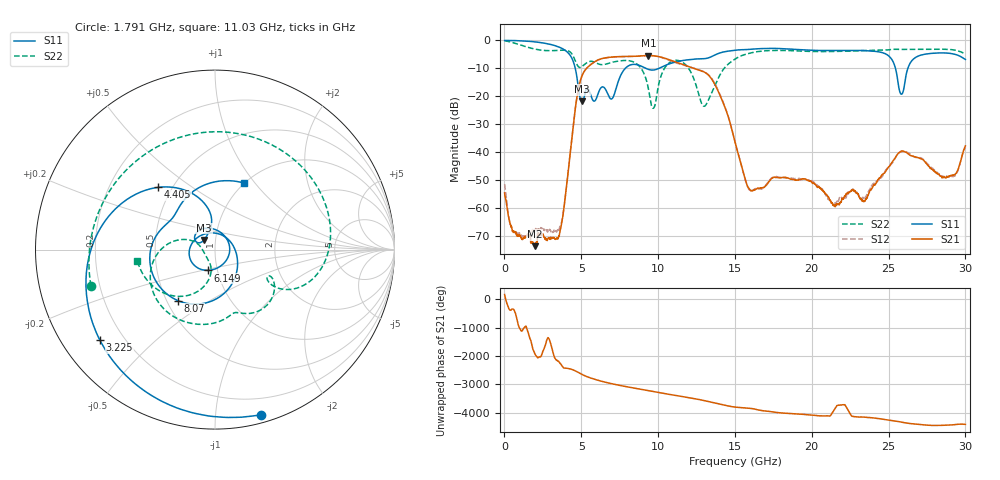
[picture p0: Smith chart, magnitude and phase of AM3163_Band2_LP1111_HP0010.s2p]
!Agilent Technologies,E8364B,MY43040894,A.07.50.67
!Agilent E8364B: A.07.50.67
!Date: Thursday, August 20, 2020 12:07:08
!Correction: S11(Full 2 Port(1,2))
!S21(Full 2 Port(1,2))
!S12(Full 2 Port(1,2))
!S22(Full 2 Port(1,2))
!S2P File: Measurements: S11, S21, S12, S22:
# Hz S  dB  R 50
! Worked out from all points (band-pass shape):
!   3201 points, 10 MHz to 30 GHz, reference 50 ohm
!   highest |S21| = -5.40 dB at 9.363 GHz (marker M1); lowest = -73.5 dB at 1.959 GHz (marker M2)
!   |S21| within 3 dB of the highest: 5.671 GHz to 11.48 GHz (5.805 GHz wide, 67.7 % of centre)
!   lowest |S11| = -21.8 dB at 5.052 GHz (marker M3), VSWR 1.18, Z = 44 + j4.75 ohm
!   |S11| at or under -10 dB: 4.61 GHz to 7.861 GHz (3.251 GHz wide, 52.1 % of centre); 9.212 GHz to 10.05 GHz (840.8 MHz wide, 8.73 % of centre); 25.45 GHz to 26.25 GHz (803.1 MHz wide, 3.11 % of centre)
!   |S22| runs from -24.3 to -0.1 dB; largest |S21 - S12| = 0.013
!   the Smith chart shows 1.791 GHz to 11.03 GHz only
!   S11 on the Smith chart (normalised r, x): 1.791 GHz: 0.06, -1.31; 3.225 GHz: 0.11, -0.34; 4.405 GHz: 0.42, +0.37; 6.149 GHz: 0.90, -0.21; 8.07 GHz: 0.57, -0.37; 11.03 GHz: 1.00, +0.88
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1e7  -0.01 -2.9  -54.48 159.8  -51.36 74.3  -0.12 -6.9
8.440969e8  -0.09 -34.6  -69.99 -70.2  -69.32 -162.8  -1.27 -82.0
1.790656e9  -0.40 -74.5  -72.08 177.6  -68.10 48.2  -2.85 -163.8
1.95935e9  -0.50 -81.8  -73.54 -103.5  -67.92 -139.6  -3.07 -177.5
3.224553e9  -1.76 -141.7  -70.62 157.8  -67.99 -81.7  -3.64 83.4
4.405409e9  -6.57 132.4  -33.92 41.6  -33.92 41.0  -4.93 -16.9
5.014581e9  -21.66 132.5  -13.11 -122.4  -13.11 -122.7  -9.48 -25.8
5.052069e9  -21.78 138.8  -12.58 -132.8  -12.59 -133.1  -9.32 -25.7
6.148578e9  -18.21 -109.5  -6.84 14.2  -6.87 14.1  -8.47 -68.9
6.982675e9  -20.90 55.3  -5.94 -97.5  -5.99 -97.7  -7.86 -88.2
8.069812e9  -9.08 -126.2  -5.75 144.4  -5.77 144.7  -7.22 -131.7
9.363131e9  -10.34 151.5  -5.40 19.3  -5.38 19.1  -17.06 159.0
1.000979e10  -10.10 128.7  -5.75 -44.5  -5.78 -45.1  -16.46 -100.4
1.103132e10  -7.86 66.4  -7.51 -140.9  -7.77 -140.5  -7.20 -171.9
1.299942e10  -6.54 -49.8  -11.29 28.6  -11.23 30.1  -23.54 -99.7
1.5005e10  -3.51 -132.8  -36.39 159.8  -36.27 159.0  -6.69 -112.2
1.787279e10  -2.90 98.0  -49.10 -38.9  -48.90 -38.4  -3.58 92.0
2.000958e10  -3.53 -9.9  -50.75 -122.5  -50.14 -119.9  -3.94 -9.6
2.230569e10  -3.57 -99.9  -54.76 111.5  -55.02 -134.2  -3.86 -93.6
2.500479e10  -5.52 158.3  -45.22 66.1  -45.12 65.2  -3.36 -167.7
2.583889e10  -19.23 171.6  -39.59 -9.8  -39.77 -9.9  -3.21 169.7
3e10  -6.80 50.9  -37.71 -87.7  -38.19 -85.1  -4.80 55.2
